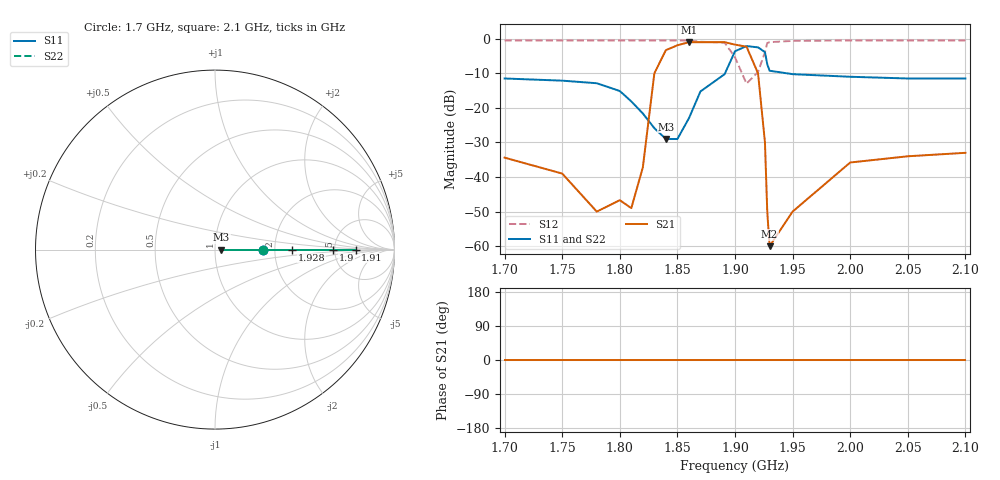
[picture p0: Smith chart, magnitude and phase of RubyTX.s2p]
# GHZ S dB R 50
!Dati letti dall'articolo di Ruby (solo S21!)
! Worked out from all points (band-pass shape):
!   22 points, 1.7 GHz to 2.1 GHz, reference 50 ohm
!   highest |S21| = -1.00 dB at 1.86 GHz (marker M1); lowest = -60.0 dB at 1.93 GHz (marker M2)
!   |S21| within 3 dB of the highest: 1.839 GHz to 1.912 GHz (73.25 MHz wide, 3.91 % of centre)
!   lowest |S11| = -29.0 dB at 1.84 GHz (marker M3), VSWR 1.07, Z = 53.7 + j0 ohm
!   |S11| at or under -10 dB: start of sweep to 1.891 GHz; 1.945 GHz to end of sweep
!   |S22| runs from -29.0 to -2.1 dB; largest |S21 - S12| = 0.94
!   S11 on the Smith chart (normalised r, x): 1.7 GHz: 1.73, +0.00; 1.9 GHz: 4.86, +0.00; 1.91 GHz: 8.22, +0.00; 1.928 GHz: 2.50, +0.00; 2.1 GHz: 1.73, +0.00
1.7  -11.50 0.0  -34.40 0.0  -0.50 0.0  -11.50 0.0
1.75  -12.12 0.0  -39.00 0.0  -0.50 0.0  -12.12 0.0
1.78  -12.88 0.0  -50.00 0.0  -0.50 0.0  -12.88 0.0
1.8  -15.12 0.0  -46.70 0.0  -0.50 0.0  -15.12 0.0
1.81  -18.12 0.0  -49.00 0.0  -0.50 0.0  -18.12 0.0
1.82  -21.62 0.0  -37.20 0.0  -0.50 0.0  -21.62 0.0
1.83  -25.88 0.0  -10.00 0.0  -0.50 0.0  -25.88 0.0
1.84  -29.00 0.0  -3.30 0.0  -0.50 0.0  -29.00 0.0
1.85  -29.00 0.0  -1.90 0.0  -0.50 0.0  -29.00 0.0
1.86  -23.00 0.0  -1.00 0.0  -0.50 0.0  -23.00 0.0
1.87  -15.25 0.0  -1.00 0.0  -0.88 0.0  -15.25 0.0
1.891  -10.25 0.0  -1.00 0.0  -1.12 0.0  -10.25 0.0
1.9  -3.62 0.0  -1.70 0.0  -5.37 0.0  -3.62 0.0
1.91  -2.12 0.0  -2.30 0.0  -13.00 0.0  -2.12 0.0
1.92  -2.50 0.0  -10.00 0.0  -9.62 0.0  -2.50 0.0
1.926  -3.88 0.0  -30.00 0.0  -3.88 0.0  -3.88 0.0
1.928  -7.38 0.0  -50.00 0.0  -1.25 0.0  -7.38 0.0
1.93  -9.25 0.0  -60.00 0.0  -1.00 0.0  -9.25 0.0
1.95  -10.25 0.0  -50.00 0.0  -0.62 0.0  -10.25 0.0
2  -11.00 0.0  -35.80 0.0  -0.50 0.0  -11.00 0.0
2.05  -11.50 0.0  -34.00 0.0  -0.50 0.0  -11.50 0.0
2.1  -11.50 0.0  -33.00 0.0  -0.50 0.0  -11.50 0.0
